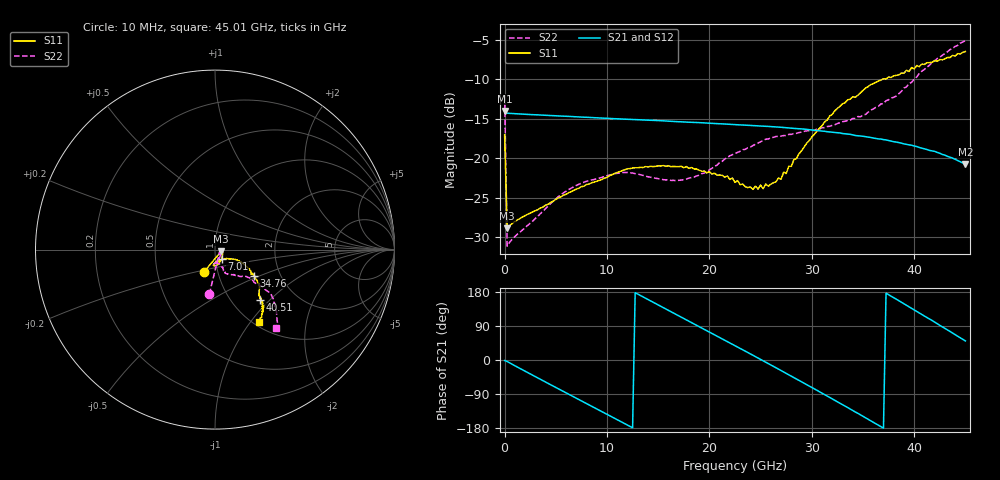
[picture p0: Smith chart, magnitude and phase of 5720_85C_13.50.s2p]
! Device:  ADRF5720
! Description: 0.5dB LSB GaAs MMIC 6-bit Digital Attenuator
! Frequency:  0.000009 -  40 GHz
! Ports:
!	RF1	= Port 1
!	RF2	= Port 2
! Vdd:  3.3 Volt
! Vss:  -3.3 Volt
! Control:  0/3.3 Volt
! State:  13.50 dB attenuation
! Data:  The device was measured using G-S-G Probes on a matrix board.
!  Data was collected using an calibrated 4 port network analyzer.
!  The reference plane for this measurement is at the launchers.
! Note:  Analog Devices supplies this data as a sample of measured data
!  for this product.  Your particular data for this product may vary.
!  Data was taken at 85 degrees C.
!  Analog Devices reserves the right to change this data at anytime.
# GHZ S DB R 45.0
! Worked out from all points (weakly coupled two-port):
!   181 points, 10 MHz to 45.01 GHz, reference 45 ohm
!   highest |S21| = -14.02 dB at 10 MHz (marker M1); lowest = -20.8 dB at 45.01 GHz (marker M2)
!   lowest |S11| = -28.9 dB at 260 MHz (marker M3), VSWR 1.07, Z = 48.2 - j0.815 ohm
!   |S11| at or under -10 dB: start of sweep to 36.94 GHz
!   |S22| runs from -31.1 to -5.1 dB; largest |S21 - S12| = 0.00094
!   S11 on the Smith chart (normalised r, x): 10 MHz: 0.86, -0.22; 7.01 GHz: 1.07, -0.11; 34.76 GHz: 1.46, -0.46; 40.51 GHz: 1.34, -0.89; 45.01 GHz: 1.05, -1.10
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0.01  -17.03 -116.5  -14.02 -1.4  -14.00 -1.4  -12.03 -97.3
0.26  -28.90 -13.6  -14.31 -4.0  -14.30 -4.0  -31.14 -17.7
3.76  -26.19 -31.6  -14.55 -54.6  -14.54 -54.6  -26.73 -51.3
7.01  -23.93 -55.2  -14.76 -100.9  -14.75 -100.8  -23.45 -77.4
7.76  -23.54 -59.0  -14.81 -111.5  -14.80 -111.4  -23.05 -81.0
11.76  -21.46 -78.9  -15.06 -168.2  -15.05 -168.1  -21.81 -95.9
15.26  -21.00 -90.8  -15.26 141.9  -15.25 142.1  -22.65 -95.9
19.01  -21.52 -94.9  -15.50 88.3  -15.49 88.5  -22.16 -77.1
22.76  -22.84 -84.7  -15.77 34.3  -15.75 34.5  -19.27 -67.5
24.76  -23.93 -70.3  -15.91 5.3  -15.90 5.5  -18.08 -67.6
27.01  -22.66 -43.3  -16.09 -27.8  -16.07 -27.6  -17.20 -66.2
27.26  -21.77 -39.6  -16.12 -31.6  -16.11 -31.3  -17.14 -66.7
27.51  -21.95 -38.1  -16.15 -35.2  -16.13 -35.0  -17.14 -65.8
27.76  -21.02 -34.8  -16.17 -38.9  -16.16 -38.6  -16.99 -66.4
28.01  -21.03 -34.8  -16.20 -42.7  -16.19 -42.4  -16.99 -65.8
30.26  -16.97 -26.6  -16.47 -76.2  -16.45 -75.9  -16.50 -63.3
33.01  -13.12 -29.4  -16.88 -118.0  -16.86 -117.8  -15.38 -55.8
34.76  -11.73 -34.1  -17.18 -144.7  -17.17 -144.4  -14.77 -51.1
37.76  -9.79 -40.7  -17.85 168.2  -17.83 168.6  -12.38 -40.2
40.51  -8.42 -48.1  -18.65 124.0  -18.63 124.4  -9.25 -37.9
42.26  -7.73 -50.5  -19.27 95.6  -19.24 96.0  -7.38 -40.3
45.01  -6.50 -59.0  -20.77 50.4  -20.74 50.8  -5.10 -52.0
